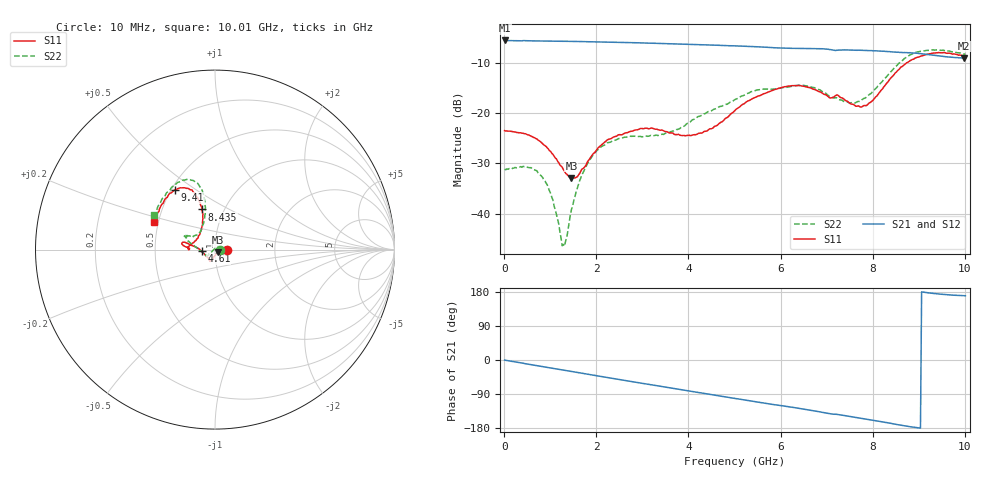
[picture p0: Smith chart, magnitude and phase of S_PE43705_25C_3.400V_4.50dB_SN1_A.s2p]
! Device ID: PE43705
! Serial: 1
! Insertion: A
! Impedance: 50 ohm
! Temp: 25C
! VDD: 3.400V
! Attenuation Step: 4.50dB
#  Hz  S  RI  R  50
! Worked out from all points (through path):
!   401 points, 10 MHz to 10.01 GHz, reference 50 ohm
!   highest |S21| = -5.52 dB at 10 MHz (marker M1); lowest = -9.0 dB at 9.985 GHz (marker M2)
!   group delay of S21, straight-line fit = 54.3 ps
!   lowest |S11| = -32.9 dB at 1.46 GHz (marker M3), VSWR 1.05, Z = 51.8 - j1.47 ohm
!   |S11| at or under -10 dB: start of sweep to 8.73 GHz
!   |S22| runs from -46.5 to -7.4 dB; largest |S21 - S12| = 0.0049
!   S11 on the Smith chart (normalised r, x): 10 MHz: 1.14, -0.00; 4.61 GHz: 0.86, -0.02; 8.435 GHz: 0.79, +0.37; 9.41 GHz: 0.52, +0.42; 10.01 GHz: 0.47, +0.17
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1e7  0.067 -0.000273  0.5298 -0.00256  0.5301 -0.0024  0.0278 1.54e-05
5.35e8  0.0593 0.0126  0.5151 -0.1032  0.5152 -0.1029  0.0236 0.0166
8.35e8  0.0485 0.0115  0.4998 -0.157  0.4998 -0.1566  0.0154 0.0169
1.01e9  0.041 0.00672  0.4871 -0.1881  0.4871 -0.1877  0.00939 0.0127
1.285e9  0.0271 -0.00451  0.4647 -0.2331  0.4648 -0.233  -0.00271 0.00412
1.36e9  0.0232 -0.00857  0.458 -0.2457  0.458 -0.2455  -0.00575 0.000723
1.46e9  0.0177 -0.0142  0.4479 -0.2614  0.4481 -0.2613  -0.0103 -0.00365
1.685e9  0.00666 -0.0268  0.4238 -0.2954  0.4239 -0.2953  -0.02 -0.0139
2.235e9  -0.0135 -0.0523  0.3543 -0.3682  0.3544 -0.3679  -0.0392 -0.0322
3.36e9  -0.0291 -0.0617  0.1798 -0.4614  0.1805 -0.461  -0.0539 -0.0273
4.01e9  -0.0467 -0.0383  0.0698 -0.4805  0.0702 -0.4799  -0.0795 -0.00858
4.61e9  -0.0745 -0.00953  -0.0308 -0.4745  -0.0294 -0.4744  -0.1102 0.016
5.01e9  -0.1057 0.014  -0.0929 -0.4583  -0.0925 -0.4585  -0.1326 0.0334
5.985e9  -0.1735 0.0412  -0.2229 -0.3862  -0.2208 -0.3866  -0.1626 0.07
6.685e9  -0.174 0.0205  -0.3022 -0.3203  -0.3019 -0.3202  -0.1627 0.079
7.76e9  -0.0937 0.0675  -0.3801 -0.1837  -0.3792 -0.1851  -0.076 0.1122
8.36e9  -0.0687 0.2038  -0.3989 -0.0956  -0.3978 -0.0972  -0.055 0.2442
8.435e9  -0.0717 0.2239  -0.3985 -0.0831  -0.398 -0.0849  -0.056 0.2659
8.86e9  -0.1223 0.3201  -0.3971 -0.0217  -0.394 -0.0243  -0.108 0.3742
9.41e9  -0.2221 0.3333  -0.3714 0.0365  -0.37 0.036  -0.209 0.3738
9.985e9  -0.3309 0.1645  -0.3483 0.0635  -0.3497 0.0632  -0.3301 0.2018
1.001e10  -0.3389 0.1548  -0.3496 0.0645  -0.3512 0.0637  -0.3377 0.1911
